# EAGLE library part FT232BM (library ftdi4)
USB UART 2nd Generation USB UART (USB <-> Serial)
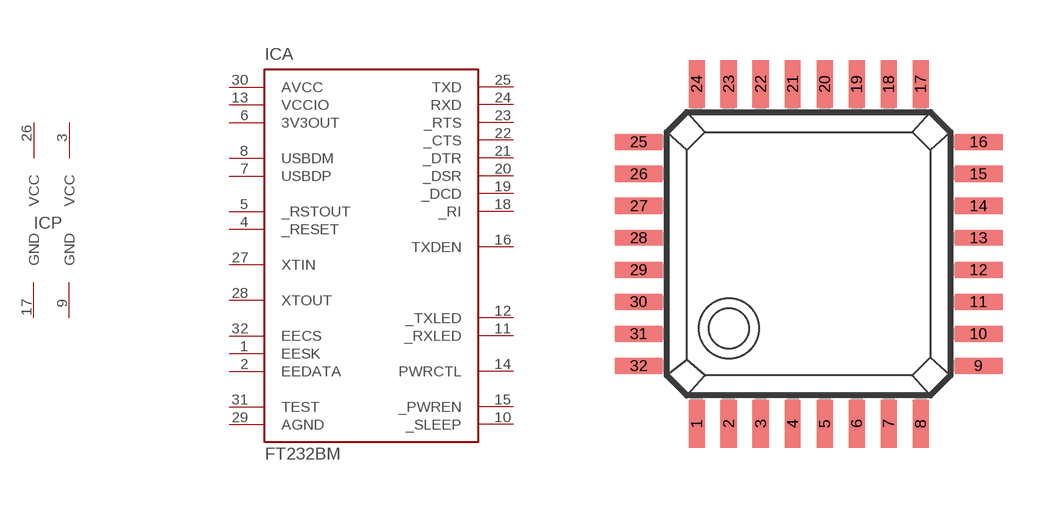
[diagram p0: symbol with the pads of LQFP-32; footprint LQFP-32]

Designator prefix IC; gates A=FT232BM P=2VCC2GND

## FT232BM  [LQFP-32]
1  A:EESK  out
2  A:EEDATA
3  P:VCC  pwr
4  A:_RESET  in
5  A:_RSTOUT  out
6  A:3V3OUT  out
7  A:USBDP
8  A:USBDM
9  P:GND  pwr
10  A:_SLEEP  out
11  A:_RXLED  oc
12  A:_TXLED  oc
13  A:VCCIO  pwr
14  A:PWRCTL  in
15  A:_PWREN  out
16  A:TXDEN  out
17  P:GND  pwr
18  A:_RI  in
19  A:_DCD  in
20  A:_DSR  in
21  A:_DTR  out
22  A:_CTS  in
23  A:_RTS  out
24  A:RXD  in
25  A:TXD  out
26  P:VCC  pwr
27  A:XTIN  in
28  A:XTOUT  out
29  A:AGND  pwr
30  A:AVCC  pwr
31  A:TEST  in
32  A:EECS

## Footprint LQFP-32 (pad centres in mm)
Quad Flat Package 32 LD LQFP Source: ds232b12.pdf http://www.ftdichip.com
smd 0.4 x 1.2: 1 -2.8,-4.25; 2 -2,-4.25; 3 -1.2,-4.25; 4 -0.4,-4.25; 5 0.4,-4.25; 6 1.2,-4.25; 7 2,-4.25; 8 2.8,-4.25; 17 2.8,4.25; 18 2,4.25; 19 1.2,4.25; 20 0.4,4.25; 21 -0.4,4.25; 22 -1.2,4.25; 23 -2,4.25; 24 -2.8,4.25
smd 1.2 x 0.4: 9 4.25,-2.8; 10 4.25,-2; 11 4.25,-1.2; 12 4.25,-0.4; 13 4.25,0.4; 14 4.25,1.2; 15 4.25,2; 16 4.25,2.8; 25 -4.25,2.8; 26 -4.25,2; 27 -4.25,1.2; 28 -4.25,0.4; 29 -4.25,-0.4; 30 -4.25,-1.2; 31 -4.25,-2; 32 -4.25,-2.8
